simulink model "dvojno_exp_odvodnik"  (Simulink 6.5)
settings: Solver=FixedStepDiscrete  StartTime=0.0  StopTime=50e-6  RelTol=1e-6
undefined symbols (not defined in the file or in its folder): blocks, Discrete, interp1, powergui, ZData
libraries: powerlib x9

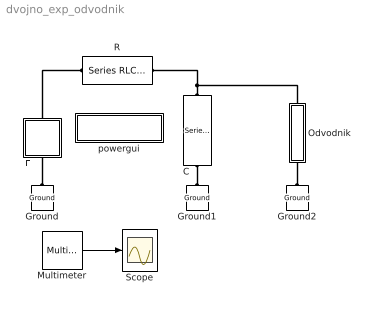
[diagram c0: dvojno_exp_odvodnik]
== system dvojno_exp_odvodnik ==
  C : powerlib/Elements/Series RLC Branch  Orientation=down  DialogController=PMDialogs.PMDefaultMaskDlg  PhysicalDomain=powersysdomain  SubClassName=unknown  LeftPortType=p1  RightPortType=p1  LConnTagsString=__new0  RConnTagsString=__new0  BranchType=C  Resistance=1  Inductance=1e-3  SetiL0=off  InitialCurrent=0  Capacitance=10e-9  Setx0=on  InitialVoltage=0  Measurements=Branch voltage
  E : Subsystem  Orientation=up  mask(Impulsen generator){UM=30e3, Tc=1.2e-6, Tz=50e-6}
      mask prompts: UM "Maksimalen napon (V)"; Tc "Vreme na celoto (s)"; Tz "Vreme na grbot (s)"
      mask help: So ovoj element e definiran idealen naponski generator so dvoen eksponencijalen oblik.
      mask init:
      | a = 0.69 / Tz;
      | b = 3.24 / Tc;
      | k = (a/b)^(-a/(a-b)) -  (a/b)^(-b/(a-b));
      | Um = UM / k;
  Ground : powerlib/Elements/Ground  Orientation=down  DialogController=PMDialogs.PMDefaultMaskDlg  PhysicalDomain=powersysdomain  SubClassName=unknown  LeftPortType=p1  RightPortType=p1  LConnTagsString=a
  Ground1 : powerlib/Elements/Ground  Orientation=down  DialogController=PMDialogs.PMDefaultMaskDlg  PhysicalDomain=powersysdomain  SubClassName=unknown  LeftPortType=p1  RightPortType=p1  LConnTagsString=a
  Ground2 : powerlib/Elements/Ground  Orientation=down  DialogController=PMDialogs.PMDefaultMaskDlg  PhysicalDomain=powersysdomain  SubClassName=unknown  LeftPortType=p1  RightPortType=p1  LConnTagsString=a
  Multimeter : powerlib/Measurements/Multimeter  SystemSampleTime=-1  PhasorSimulation=off  OutputType=Complex  sel=[2 1]  L=3  Gain=[1 1]  yselected={'Usrc: E/Kontrolirano E','Ub: C'};  PSBOutputType=1  PSBequivalent=0  AxesSetting=[0,0.1,-100,100]  Display=0  SavedBlockNames=-11
  Odvodnik : Subsystem  Orientation=up  mask(ZnO odvodnik){napon=[0	8	8.5	9	9.5	10	10.5	11	11.5	12	12.5	13]*1000, struja=[0	0	0.003	0.05	0.3	1	2.7	5.8	12.4	25.6	51.3	100]*1000}
      mask prompts: napon "Napon (V)"; struja "Struja (A)"
      mask help: So ovoj element e definiran ZnO odnodnik na prenaponi cija sto U-I karakteristika e definirana so pomos na dva vektori. Vo prviot vektor se dadeni diskretni vrednosti na naponite dodeka vrednostite na strujata za soodvetnite vrednosti na naponite se dadeni vo vtoriot vektor. Za ostanatite tocki od karakteristikata koi sto ne se dadeni vo vektorite modelot pravi linearna interpolacija.
  R : powerlib/Elements/Series RLC Branch  DialogController=PMDialogs.PMDefaultMaskDlg  PhysicalDomain=powersysdomain  SubClassName=unknown  LeftPortType=p1  RightPortType=p1  LConnTagsString=__new0  RConnTagsString=__new0  BranchType=R  Resistance=100  Inductance=1e-3  SetiL0=on  InitialCurrent=0  Capacitance=1e-6  Setx0=off  InitialVoltage=0  Measurements=None
  Scope : Scope
  powergui : Subsystem  AncestorBlock=powerlib/powergui  InitFcn=powergui( 'InitFcn_Callback' , gcb , 0 , [ ] );  mask(PSB option menu block){SimulationMode=Discrete, SampleTime=0.05e-6, echomessages=off, RestoreLinks=warning, x0status=blocks, Frange=[0:2:500], Ylog=off, Xlog=on, ShowGrid=off, save=off, variable=ZData, structure=, ZoomFFT=on, StartTime=0.0, cycles=1, DisplayStyle=1, fundamental=60, FreqAxis=off, MaxFrequency=1000, frequencyindice=0, frequencyindicesteady=1, RmsSteady=1, display=off, Ts=0, frequency=60, methode=off, HookPort=off, Interpol=off}
      mask prompts: SimulationMode "Simulation mode"; SampleTime "Sample time Ts (when simulation mode is Discrete) (s)"; echomessages "Echo  Messages"; RestoreLinks "Restore disabled links"; x0status "Initial electrical states status"; Frange "Impedance tool: Frequency Range"; Ylog "Impedance tool: Log impedance"; Xlog "Impedance tool: log Frequency"; ShowGrid "Impedance tool: grid"; save "Impedance tool: Save Data To Workspace"; variable "Impedance tool: Variable Name"; structure "Structure Name (PSBFFTSCOPE)"; ZoomFFT "ZoomFFT (PSBFFTSCOPE)"; StartTime "Start Time (PSBFFTSCOPE)"; cycles "Cycles (PSBFFTSCOPE)"; DisplayStyle "Display style (PSBFFTSCOPE)"; fundamental "Fundamental (PSBFFTSCOPE)"; FreqAxis "Frequency Axis (PSBFFTSCOPE)"; MaxFrequency "Max Frequency (PSBFFTSCOPE)"; frequencyindice "Load flow frequency (Hz)"; frequencyindicesteady "Frequency indice (STEADYSTATE)"; RmsSteady "RMS display (STEADYSTATE)"; display "Display Results"; Ts "OBSOLETE 1"; frequency "Phasor frequency (Hz)"; methode "Phasor simulation"; HookPort "Hook port"; Interpol "Interpolate"
      mask init:
      | powerlibroot = which('powersysdomain');
      | PSBroot = powerlibroot(1:end-16);
      | %
      | switch SimulationMode
      | 	case 1
      | 		message=sprintf('Continuous');
      | 	case 2
      |         SampleTimeeval=evalin('base',SampleTime,'NaN');
      |         if isnan(SampleTimeeval)
      |             message=sprintf('Warning !!,\nUndefined sample time');
      |         else
      |             message=sprintf('Discrete,\nTs = %.4g s.',SampleTimeeval);
      |         end
      | 	case 3
      | 		message=sprintf('Phasors');
      | end
      | if strcmp(bdroot,'powerlib')
      |   message='powergui';
      | end
      | power_initmask();
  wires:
  Multimeter/1 -> Scope/1
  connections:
  C/LConn1 -- R/RConn1 -- Odvodnik/RConn1
  Ground1/LConn1 -- C/RConn1
  Ground/LConn1 -- E/LConn1
  E/RConn1 -- R/LConn1
  Odvodnik/LConn1 -- Ground2/LConn1

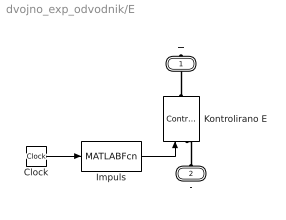
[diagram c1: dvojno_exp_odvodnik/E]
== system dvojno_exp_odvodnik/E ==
  Clock : Clock
  Impuls : MATLABFcn  MATLABFcn=Um*(exp(-a*u)-exp(-b*u))  OutputSignalType=real
  Kontrolirano E : powerlib/Electrical Sources/Controlled Voltage Source  Orientation=up  DialogController=PMDialogs.PMDefaultMaskDlg  SystemSampleTime=-1  Initialize=on  Source_Type=AC  Amplitude=0  Phase=0  Frequency=0  Measurements=Voltage
  + : PMIOPort  Orientation=down  Port=1  Side=Right
  - : PMIOPort  Orientation=up  Port=2  Side=Left
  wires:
  Impuls/1 -> Kontrolirano E/1
  Clock/1 -> Impuls/1
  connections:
  +/RConn1 -- Kontrolirano E/RConn1
  -/RConn1 -- Kontrolirano E/LConn1

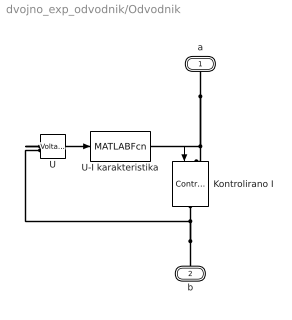
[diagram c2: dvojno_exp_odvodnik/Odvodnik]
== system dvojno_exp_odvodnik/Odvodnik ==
  Kontrolirano I : powerlib/Electrical Sources/Controlled Current Source  Orientation=down  DialogController=PMDialogs.PMDefaultMaskDlg  SystemSampleTime=-1  Initialize=on  Source_Type=AC  Amplitude=0  Phase=0  Frequency=0  Measurements=Current
  U : powerlib/Measurements/Voltage Measurement  DialogController=PMDialogs.PMDefaultMaskDlg  SystemSampleTime=-1  PhasorSimulation=off  OutputType=Complex  PSBequivalent=0
  U-I karakteristika : MATLABFcn  MATLABFcn=interp1(napon, struja, u)  OutputSignalType=real
  a : PMIOPort  Orientation=down  Port=1  Side=Right
  b : PMIOPort  Orientation=up  Port=2  Side=Left
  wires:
  U/1 -> U-I karakteristika/1
  U-I karakteristika/1 -> Kontrolirano I/1
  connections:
  Kontrolirano I/LConn1 -- a/RConn1 -- U/LConn1
  Kontrolirano I/RConn1 -- b/RConn1 -- U/LConn2

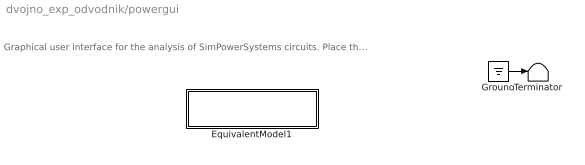
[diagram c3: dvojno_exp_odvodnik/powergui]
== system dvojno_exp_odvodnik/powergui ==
  note: Graphical user interface for the analysis of SimPowerSystems circuits. Place the Powergui block in the top-level of your model and double-click on it to open the GUI.
  EquivalentModel1 : Subsystem
  Ground : Ground
  Terminator : Terminator
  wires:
  Ground/1 -> Terminator/1

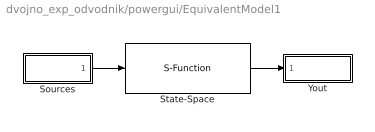
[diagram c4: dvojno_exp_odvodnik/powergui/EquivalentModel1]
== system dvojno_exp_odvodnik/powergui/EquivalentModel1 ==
  Sources : Subsystem
  State-Space : S-Function  FunctionName=sfun_spssw_discc  Parameters=Ts,A, B, C, D, x0
  Yout : Subsystem
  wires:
  Sources/1(u) -> State-Space/1
  State-Space/1 -> Yout/1(v,i)

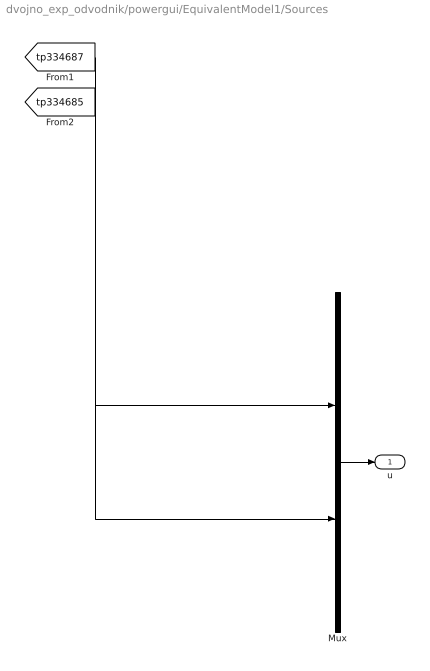
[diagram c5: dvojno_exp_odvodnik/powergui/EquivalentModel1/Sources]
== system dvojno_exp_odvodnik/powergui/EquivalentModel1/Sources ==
  Mux : Mux  Inputs=[1 1]
  u : Outport
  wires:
  Mux/1 -> u/1
  [tp334687] -> Mux/1
  [tp334685] -> Mux/2

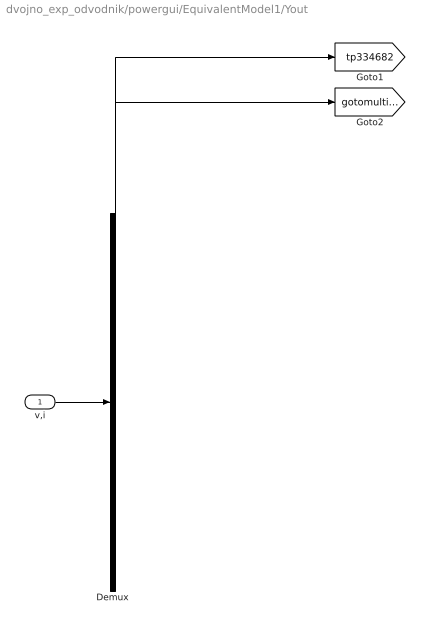
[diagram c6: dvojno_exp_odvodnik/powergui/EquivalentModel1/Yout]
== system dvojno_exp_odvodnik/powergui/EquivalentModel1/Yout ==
  v,i : Inport
  Demux : Demux  Outputs=[1 3]
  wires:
  v,i/1 -> Demux/1
  Demux/1 -> [tp334682]
  Demux/2 -> [gotomultimeterPSB]
